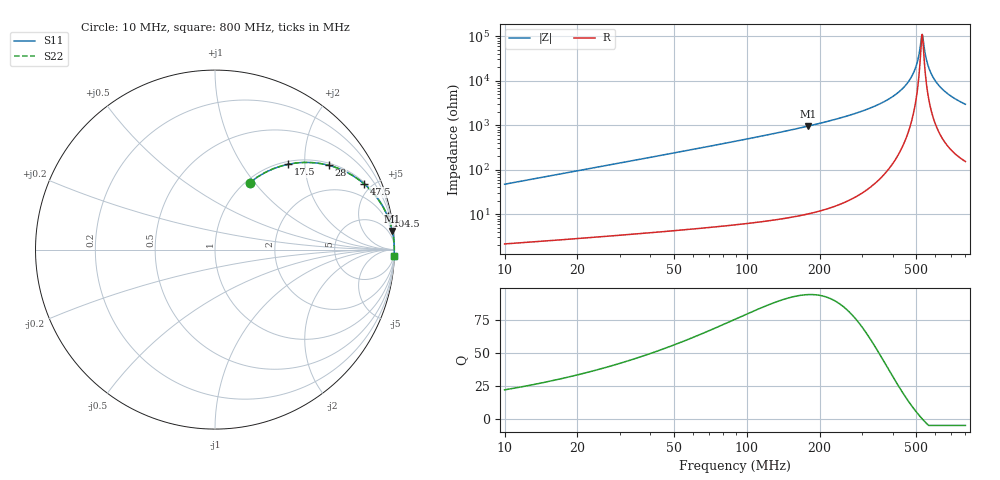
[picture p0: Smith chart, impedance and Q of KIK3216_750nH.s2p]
!version-2
!date-01.2022
!Series
# MHz S RI R 50
!Freq ReS11 ImS11 ReS21 ImS21 ReS12 ImS12 ReS22 ImS22
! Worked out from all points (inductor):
!   528 points, 10 MHz to 800 MHz, reference 50 ohm
!   read as one part in series: L = 750 nH near 13 MHz
!   highest Q = 94 at 179.5 MHz (marker M1), where L = 847 nH
!   self-resonance near 529 MHz
!   S11 on the Smith chart (normalised r, x): 10 MHz: 1.04, +0.94; 17.5 MHz: 1.05, +1.65; 28 MHz: 1.07, +2.65; 47.5 MHz: 1.08, +4.51; 104.5 MHz: 1, +10; 800 MHz: 4, -59
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10  0.1929 0.3725  0.8071 -0.3725  0.8071 -0.3725  0.1929 0.3725
17.5  0.4085 0.4756  0.5915 -0.4756  0.5915 -0.4756  0.4085 0.4756
28  0.6334 0.4697  0.3666 -0.4697  0.3666 -0.4697  0.6334 0.4697
47.5  0.8314 0.3653  0.1686 -0.3653  0.1686 -0.3653  0.8314 0.3653
70  0.9151 0.2713  0.0849 -0.2713  0.0849 -0.2713  0.9151 0.2713
104.5  0.9612 0.1871  0.0388 -0.1871  0.0388 -0.1871  0.9612 0.1871
142  0.9797 0.1357  0.0203 -0.1357  0.0203 -0.1357  0.9797 0.1357
179.5  0.9881 0.1033  0.0119 -0.1033  0.0119 -0.1033  0.9881 0.1033
274  0.9961 0.0565  0.00393 -0.0565  0.00393 -0.0565  0.9961 0.0565
406  0.9988 0.0216  0.00118 -0.0216  0.00118 -0.0216  0.9988 0.0216
455.5  0.9991 0.0122  0.000924 -0.0122  0.000924 -0.0122  0.9991 0.0122
490  0.9991 0.00634  0.000873 -0.00634  0.000873 -0.00634  0.9991 0.00634
511  0.9991 0.00298  0.000882 -0.00298  0.000882 -0.00298  0.9991 0.00298
529  0.9991 0.000217  0.000911 -0.000217  0.000911 -0.000217  0.9991 0.000217
533.5  0.9991 -0.00046  0.000921 0.00046  0.000921 0.00046  0.9991 -0.00046
538  0.9991 -0.00113  0.000932 0.00113  0.000932 0.00113  0.9991 -0.00113
545.5  0.999 -0.00224  0.000953 0.00224  0.000953 0.00224  0.999 -0.00224
554.5  0.999 -0.00354  0.000981 0.00354  0.000981 0.00354  0.999 -0.00354
578.5  0.9989 -0.00693  0.00108 0.00693  0.00108 0.00693  0.9989 -0.00693
616  0.9987 -0.012  0.00127 0.012  0.00127 0.012  0.9987 -0.012
668.5  0.9984 -0.0186  0.00163 0.0186  0.00163 0.0186  0.9984 -0.0186
800  0.9971 -0.0336  0.00288 0.0336  0.00288 0.0336  0.9971 -0.0336
